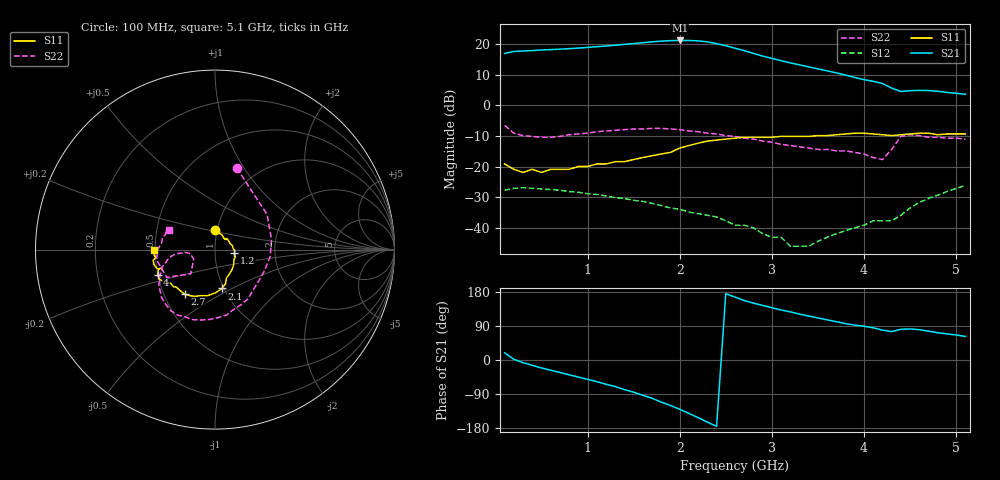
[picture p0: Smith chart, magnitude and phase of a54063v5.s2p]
!  INA-54063 S PARAMETERS
!  Vd = 5 V  Id = 30 mA  LAST UPDATED 10-07-96
# ghz s ma r 50
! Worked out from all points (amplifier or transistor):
!   51 points, 100 MHz to 5.1 GHz, reference 50 ohm
!   highest |S21| = 21.2 dB at 2 GHz (marker M1)
!   |S21| within 3 dB of that: 590 MHz to 2.658 GHz (2.068 GHz wide, 127 % of centre)
!   unconditionally stable (mu >= 1): start of sweep to end of sweep
!   at 900 MHz: K = 1.47, MAG = 19.5 dB, |S12| = -28.4 dB
!   at 2.6 GHz: K = 4.41, MAG = 19.5 dB, |S12| = -39.2 dB
!   at 5.1 GHz: K = 5.63, MAG = 4.4 dB, |S12| = -26.2 dB
!   S11 on the Smith chart (normalised r, x): 100 MHz: 0.97, +0.22; 1.2 GHz: 1.24, -0.05; 2.1 GHz: 0.98, -0.45; 2.7 GHz: 0.64, -0.35; 4 GHz: 0.50, -0.16; 5.1 GHz: 0.49, +0.00
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0.1  0.11 91.0  7.02 19.0  0.041 21.0  0.47 75.0
0.2  0.09 64.0  7.56 2.0  0.044 7.0  0.35 34.0
0.5  0.08 46.0  8 -21.0  0.043 -9.0  0.3 -23.0
1  0.1 5.0  8.8 -51.0  0.036 -21.0  0.35 -73.0
1.2  0.11 -11.0  9.28 -64.0  0.033 -25.0  0.38 -88.0
1.3  0.12 -20.0  9.58 -70.0  0.031 -26.0  0.39 -94.0
1.5  0.13 -36.0  10.19 -85.0  0.028 -28.0  0.41 -108.0
1.7  0.15 -53.0  10.86 -101.0  0.025 -30.0  0.42 -120.0
1.8  0.16 -61.0  11.16 -111.0  0.023 -31.0  0.42 -126.0
2  0.2 -73.0  11.44 -130.0  0.02 -29.0  0.4 -138.0
2.1  0.22 -80.0  11.43 -141.0  0.018 -29.0  0.38 -144.0
2.2  0.24 -89.0  11.25 -152.0  0.017 -28.0  0.37 -148.0
2.3  0.26 -99.0  10.86 -164.0  0.016 -27.0  0.35 -151.0
2.5  0.28 -112.0  9.39 175.0  0.013 -24.0  0.32 -158.0
2.6  0.29 -117.0  8.55 166.0  0.011 -23.0  0.31 -162.0
2.7  0.3 -124.0  7.79 157.0  0.011 -15.0  0.29 -164.0
3.1  0.31 -138.0  5.35 132.0  0.007 3.0  0.23 -173.0
3.5  0.32 -145.0  3.93 111.0  0.006 65.0  0.19 -174.0
4  0.35 -156.0  2.62 89.0  0.011 99.0  0.16 -174.0
4.3  0.32 -161.0  1.91 75.0  0.013 112.0  0.19 -135.0
4.5  0.34 -162.0  1.73 82.0  0.021 129.0  0.33 -170.0
5.1  0.34 180.0  1.51 62.0  0.049 120.0  0.28 157.0
